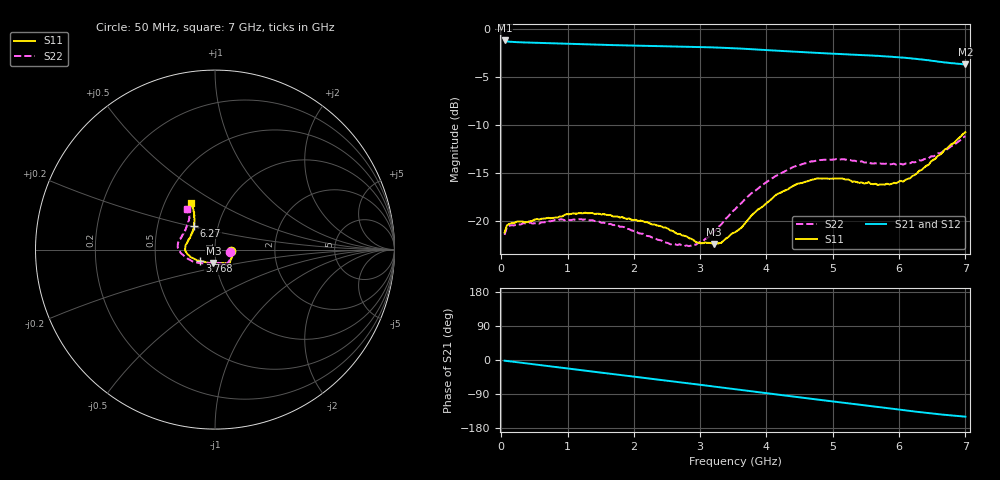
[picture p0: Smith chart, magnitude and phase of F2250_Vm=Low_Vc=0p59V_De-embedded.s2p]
! Integrated Device Technology
! Corporate Headquarters
! 6024 Silver Creek Valley Road
! San Jose, CA 95138  USA
! Phone:  1-408-284-8200
! Toll Free:  1-800-223-1366
! Webpage:  http://www.idt.com/
! Timing and RF Division
! 515 Groton Road, Suite 102
! Westford, MA 01886-6024
! Device:  F2250
! Description: Voltage Variable RF Attenuator
! Frequency:  50.0 -  6000.00 MHz
! Package:  3x3 mm Thin QFN Plastic Package: 16 pin
! Ports:  2 RF, 3 DC
!  Pin  1  = GND
!  Pin  2  = NC
!  Pin  3  = RF1  = Port 1
!  Pin  4  = NC
!  Pin  5  = GND
!  Pin  6  = GND
!  Pin  7  = GND
!  Pin  8  = GND
!  Pin  9  = NC
!  Pin 10  = RF2  = Port 2
!  Pin 11  = NC
!  Pin 12  = GND
!  Pin 13  = GND
!  Pin 14  = VCNTRL
!  Pin 15  = VDD
!  Pin 16  = VMODE
! Vcntrl:  0.590 Volts
! Vmode:  +0.000 Volts
! Vdd:  +3.30  Volts
! Current:  1.137 mA
! Data:  The device was measured on a the F2250 evaluation board which has
!  individual transmission lines to the RF pins.  Data was collected
!  using a calibrated network analyzer.  The evaluation board was
!  de-embedded using a TRL calibration technique.
!  The reference plane is the edge of the package pin.
! Misc:  SN 10
!  Action Tracker AT0258
! Date Measured:  2014-11-26
! Date:  2015-10-15  MJV
! Note:
!  Integrated Device Technology supplies this data as a sample of measured
!  data at the package pin for this product.  Your particular data for this
!  product may vary.
!  Data was taken at 25 degrees C.
!  Integrated Device Technology reserves the right to change this data at anytime.
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# GHz S dB R 50
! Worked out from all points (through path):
!   201 points, 50 MHz to 7 GHz, reference 50 ohm
!   highest |S21| = -1.24 dB at 50 MHz (marker M1); lowest = -3.7 dB at 7 GHz (marker M2)
!   group delay of S21, straight-line fit = 60.1 ps
!   lowest |S11| = -22.4 dB at 3.212 GHz (marker M3), VSWR 1.16, Z = 48.5 - j7.34 ohm
!   |S11| at or under -10 dB: start of sweep to end of sweep
!   |S22| runs from -22.6 to -11.2 dB; largest |S21 - S12| = 0.00042
!   S11 on the Smith chart (normalised r, x): 50 MHz: 1.19, -0.02; 3.768 GHz: 0.84, -0.11; 6.27 GHz: 0.77, +0.21; 7 GHz: 0.68, +0.38
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0.05  -21.21 -6.2  -1.24 -1.8  -1.23 -1.8  -21.43 -7.4
0.08475  -20.45 -6.5  -1.33 -2.5  -1.33 -2.5  -20.63 -7.0
0.15425  -20.22 -8.4  -1.38 -4.0  -1.38 -4.0  -20.43 -8.9
0.71025  -19.66 -29.4  -1.52 -16.2  -1.51 -16.2  -20.00 -33.2
1.2315  -19.19 -44.8  -1.64 -27.4  -1.63 -27.4  -19.85 -52.8
1.75275  -19.53 -51.6  -1.73 -38.5  -1.73 -38.5  -20.39 -62.6
2.37825  -20.50 -54.4  -1.82 -51.8  -1.82 -51.8  -21.98 -71.3
2.83  -21.77 -67.9  -1.89 -61.7  -1.88 -61.7  -22.61 -92.6
3.0385  -22.30 -82.5  -1.92 -66.3  -1.92 -66.3  -22.09 -107.8
3.21225  -22.41 -96.9  -1.96 -70.2  -1.96 -70.2  -21.10 -120.8
3.3165  -22.27 -107.7  -1.99 -72.5  -1.99 -72.5  -20.36 -127.6
3.525  -21.17 -125.8  -2.05 -77.2  -2.05 -77.2  -18.79 -139.7
3.76825  -19.46 -143.7  -2.14 -82.6  -2.14 -82.6  -17.13 -151.0
4.1505  -17.24 -160.7  -2.30 -91.0  -2.30 -91.0  -15.28 -166.8
4.46325  -16.13 -170.6  -2.42 -97.7  -2.42 -97.7  -14.25 -175.6
4.7065  -15.68 -177.4  -2.51 -103.0  -2.51 -103.0  -13.80 178.9
5.15825  -15.61 171.5  -2.67 -112.7  -2.67 -112.7  -13.57 169.1
5.85325  -16.19 147.7  -2.91 -127.6  -2.92 -127.6  -14.12 153.3
6.06175  -15.90 139.5  -3.02 -132.1  -3.02 -132.2  -14.14 147.2
6.27025  -15.03 131.2  -3.16 -136.7  -3.16 -136.7  -13.83 140.7
6.61775  -13.11 120.9  -3.46 -143.4  -3.46 -143.4  -12.95 129.0
7  -10.77 117.3  -3.73 -149.5  -3.73 -149.6  -11.17 124.8
